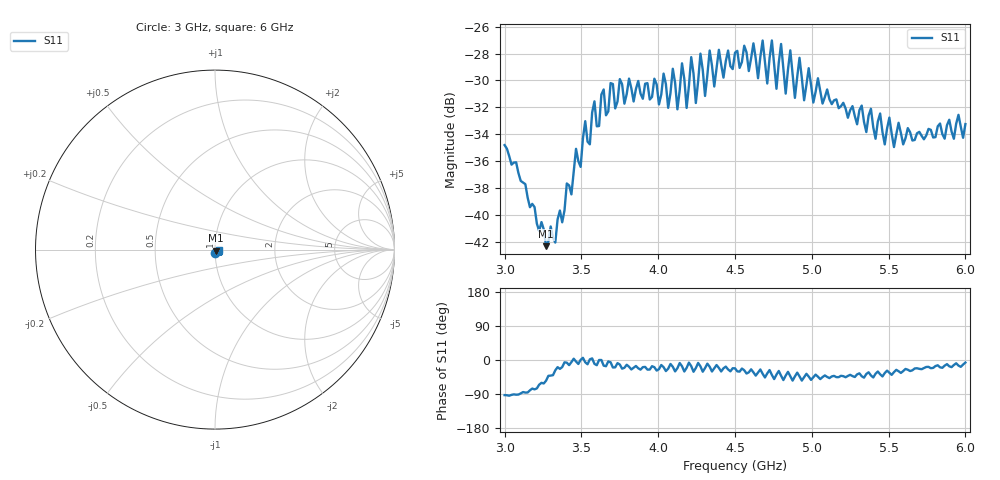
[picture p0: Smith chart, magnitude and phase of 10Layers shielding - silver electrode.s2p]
!  03/07/2025  17:29:33
! Ref Plane: 0.000 mm
# MHZ S MA R  50
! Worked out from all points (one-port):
!   201 points, 3 GHz to 6 GHz, reference 50 ohm
!   lowest |S11| = -42.3 dB at 3.27 GHz (marker M1), VSWR 1.02, Z = 50.4 - j0.628 ohm
!   |S11| at or under -10 dB: start of sweep to end of sweep
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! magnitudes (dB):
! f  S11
! 3 GHz  -34.8
! 3.27 GHz  -42.3
! 3.375 GHz  -40.6
! 3.525 GHz  -33.0
! 3.555 GHz  -34.8
! 3.585 GHz  -31.6
! 3.615 GHz  -33.4
! 3.75 GHz  -29.9
! 4.005 GHz  -31.8
! 4.035 GHz  -29.5
! 4.065 GHz  -32.0
! 4.095 GHz  -29.1
! 4.125 GHz  -32.1
! 4.155 GHz  -28.7
! 4.185 GHz  -32.0
! 4.215 GHz  -28.3
! 4.245 GHz  -31.7
! 4.275 GHz  -28.0
! 4.305 GHz  -31.2
! 4.335 GHz  -27.8
! 4.365 GHz  -30.4
! 4.395 GHz  -27.7
! 4.425 GHz  -29.8
! 4.5 GHz  -27.9
! 4.875 GHz  -29.5
! 5.25 GHz  -32.2
! 5.625 GHz  -33.5
! 6 GHz  -33.2
